[IBIS Ver]   4.2
[File Name]  stm32f2_ufbga176.ibs
[File Rev]   1.0
[Date]   31-Aug-2011
[Source]   STMicroelectronics NV
[Notes]   The I/O models have been made by simulation and qualified
   with recomandation of QualityIBIS flow.
   Some Models, library and pin names may be modified.
   Details of modified names can be found below.
ORIGINAL NAME   ::  MODIFIED NAME   :: COMMENTS(if any)
IO8USB_LSFS_OTG_FT  ::  IO8USB_LSFS_OTG_FT_USB   :: Model in USB mode.
IO8USB_LSFS_OTG_FT  ::  IO8USB_LSFS_OTG_FT_NON_USB_DNV33  :: Model in other than USB mode & pad pin = DNV33
IO8USB_LSFS_OTG_FT  ::  IO8USB_LSFS_OTG_FT_NON_USB_DPV33  :: Model in other than USB mode & pad pin = DPV33
[Disclaimer] These IBIS models are the proprietary information of
   STMicroelectronics and are disclosed to users solely for
   modeling and simulation purposes. No further license is
   implied. All warranties express, implied, or statutory,
   including any implied warranty of fitness for a particular
   purpose or implied warranty against infringement, are
   hereby disclaimed. STMicroelectronics reserves the right
   to change the IBIS models at any time and without notice.
[Copyright]  (c) STMicroelectronics
   All rights reserved. Reproduction in whole or part is prohibited
   without the written consent of the copyright holder.
[Component]  STM32F2_UFBGA176
[Manufacturer] STMicroelectronics NV
[Package]
| variable   typ   min   max
R_pkg   0.000mOhm   0.000mOhm   0.000mOhm
L_pkg   0.000nH   0.000nH   0.000nH
C_pkg   0.000pF   0.000pF   0.000pF
[Pin]   signal_name   model_name
A2 PE2 IO8PROG2M25M50M100M_ARSUDQ_FT
A1 PE3 IO8PROG2M25M50M100M_ARSUDQ_FT
B1 PE4 IO8PROG2M25M50M100M_ARSUDQ_FT
B2 PE5 IO8PROG2M25M50M100M_ARSUDQ_FT
B3 PE6 IO8PROG2M25M50M100M_ARSUDQ_FT
|C1 VBAT VDD33IOSWCO_MOSSWI_FT
D2 PI8 IO8PROG2M25M50M100M_ARSUDQ_FT_V33
D1 PC13 IO8PROG2M25M50M100M_ARWSUDQ_FT_V33
E1 PC14 IO8PROG2M25M50M100M_ARWSUDQ_FT
F1 PC15 IO8PROG2M25M50M100M_ARSUDQ_FT
D3 PI9  IO8PROG2M25M50M100M_ARSUDQ_FT
E3 PI10 IO8PROG2M25M50M100M_ARSUDQ_FT
E4 PI11 IO8PROG2M25M50M100M_ARSUDQ_FT
|F2 VSS_13 VSSIOCO
|F3 VDD_13 VDD33IOCO
E2 PF0 IO8PROG2M25M50M100M_ARSUDQ_FT
H3 PF1 IO8PROG2M25M50M100M_ARSUDQ_FT
H2 PF2 IO8PROG2M25M50M100M_ARSUDQ_FT
J2 PF3 IO8PROG2M25M50M100M_ARSUDQ_FT
J3 PF4 IO8PROG2M25M50M100M_ARSUDQ_FT
K3 PF5 IO8PROG2M25M50M100M_ARSUDQ_FT
|G2 VSS_5 VSSIOCO
|G3 VDD_5 VDD33IOCO
K2 PF6 IO8PROG2M25M50M100M_ARSUDQ_FT
K1 PF7 IO8PROG2M25M50M100M_ARSUDQ_FT
L3 PF8 IO8PROG2M25M50M100M_ARSUDQ_FT
L2 PF9  IO8PROG2M25M50M100M_AR3WSUDQ_FT
L1 PF10 IO8PROG2M25M50M100M_ARSUDQ_FT
G1 PH0 IO8PROG2M25M50M100M_ARSUDQ_FT
H1 PH1 IO8PROG2M25M50M100M_ARSUDQ_FT
|J1 NRST RESET
M2 PC0 IO8PROG2M25M50M100M_AR3WSUDQ_FT
M3 PC1 IO8PROG2M25M50M100M_AR3WSUDQ_FT
M4 PC2 IO8PROG2M25M50M100M_AR3WSUDQ_FT
M5 PC3 IO8PROG2M25M50M100M_AR3WSUDQ_FT
|- VDD_12 VDD33IOCO_VSSIOCO_MOSSWI_FT
|M1 VSSA VSSCO
|N1 VREF- VSSC0
|P1 VREF+ VDD33CO
|R1 VDDA VDD33CO
N3 PA0 IO8PROG2M25M50M100M_AR3WSUDQ_FT_V33
N2 PA1 IO8PROG2M25M50M100M_AR3WSUDQ_FT
P2 PA2 IO8PROG2M25M50M100M_AR3WSUDQ_FT
F4 PH2 IO8PROG2M25M50M100M_AR3WSUDQ_FT
G4 PH3 IO8PROG2M25M50M100M_AR3WSUDQ_FT
H4 PH4 IO8PROG2M25M50M100M_AR3WSUDQ_FT
J4 PH5 IO8PROG2M25M50M100M_AR3WSUDQ_FT
R2 PA3 IO8PROG2M25M50M100M_AR3WSUDQ_FT
|- VSS_4 VSSIOCO
|L4 REGOFF   TBD
|K4 VDD_4 VDD33IOCO
N4 PA4 IO8PROG2M25M50M100M_AR3WSUDQ_FT
P4 PA5 IO8PROG2M25M50M100M_AR3WSUDQ_FT
P3 PA6 IO8PROG2M25M50M100M_AR3WSUDQ_FT
R3 PA7 IO8PROG2M25M50M100M_AR3WSUDQ_FT
N5 PC4 IO8PROG2M25M50M100M_AR3WSUDQ_FT
P5 PC5 IO8PROG2M25M50M100M_AR3WSUDQ_FT
R5 PB0 IO8PROG2M25M50M100M_AR3WSUDQ_FT
R4 PB1 IO8PROG2M25M50M100M_AR3WSUDQ_FT
M6 PB2 IO8PROG2M25M50M100M_AR3WSUDQ_FT
R6 PF11 IO8PROG2M25M50M100M_ARSUDQ_FT
P6 PF12 IO8PROG2M25M50M100M_ARSUDQ_FT
|M8 VSS_6 VSSIOCO
|N8 VDD_6 VDD33IOCO
N6 PF13 IO8PROG2M25M50M100M_ARSUDQ_FT
R7 PF14 IO8PROG2M25M50M100M_ARSUDQ_FT
P7 PF15 IO8PROG2M25M50M100M_ARSUDQ_FT
N7 PG0 IO8PROG2M25M50M100M_ARSUDQ_FT
M7 PG1 IO8PROG2M25M50M100M_ARSUDQ_FT
R8 PE7 IO8PROG2M25M50M100M_ARSUDQ_FT
P8 PE8 IO8PROG2M25M50M100M_ARSUDQ_FT
P9 PE9 IO8PROG2M25M50M100M_ARSUDQ_FT
|M9 VSS_7 VSSIOCO
|N9 VDD_7 VDD33IOCO
R9 PE10 IO8PROG2M25M50M100M_ARSUDQ_FT
P10 PE11 IO8PROG2M25M50M100M_ARSUDQ_FT
R10 PE12 IO8PROG2M25M50M100M_ARSUDQ_FT
N11 PE13 IO8PROG2M25M50M100M_ARSUDQ_FT
P11 PE14 IO8PROG2M25M50M100M_ARSUDQ_FT
R11 PE15 IO8PROG2M25M50M100M_ARSUDQ_FT
R12 PB10 IO8PROG2M25M50M100M_ARSUDQ_I2CIN_FT
R13 PB11 IO8PROG2M25M50M100M_ARSUDQ_I2CIN_FT
|M10 VCAP_1
|N10 VDD_1 VDD33IOCO
M11 PH6 IO8PROG2M25M50M100M_ARSUDQ_FT
N12 PH7 IO8PROG2M25M50M100M_ARSUDQ_FT
M12 PH8 IO8PROG2M25M50M100M_ARSUDQ_FT
M13 PH9 IO8PROG2M25M50M100M_ARSUDQ_FT
L13 PH10 IO8PROG2M25M50M100M_ARSUDQ_FT
L12 PH11 IO8PROG2M25M50M100M_ARSUDQ_FT
K12 PH12 IO8PROG2M25M50M100M_ARSUDQ_FT
|H12 VSS_14 VSSIOCO
|J12 VDD_14 VDD33IOCO
P12 PB12 IO8USB_ID_OTG_FT
P13 PB13 IO8USB_VBUS_OTG_FT
R14 PB14 IO8USB_LSFS_OTG_FT_USB
|R14 PB14 IO8USB_LSFS_OTG_FT_NON_USB_DNV33
R15 PB15 IO8USB_LSFS_OTG_FT_USB
|R15 PB15 IO8USB_LSFS_OTG_FT_NON_USB_DPV3394
P15 PD8 IO8PROG2M25M50M100M_ARSUDQ_FT
P14 PD9 IO8PROG2M25M50M100M_ARSUDQ_FT
N15 PD10 IO8PROG2M25M50M100M_ARSUDQ_FT
N14 PD11 IO8PROG2M25M50M100M_ARSUDQ_FT
N13 PD12 IO8PROG2M25M50M100M_ARSUDQ_FT
M15 PD13 IO8PROG2M25M50M100M_ARSUDQ_FT
|- VSS_8 VSSIOCO
|J13 VDD_8 VDD33IOCO
M14 PD14 IO8PROG2M25M50M100M_ARSUDQ_FT
L14 PD15 IO8PROG2M25M50M100M_ARSUDQ_FT
L15 PG2 IO8PROG2M25M50M100M_ARSUDQ_FT
K15 PG3 IO8PROG2M25M50M100M_ARSUDQ_FT
K14 PG4 IO8PROG2M25M50M100M_ARSUDQ_FT
K13 PG5 IO8PROG2M25M50M100M_ARSUDQ_FT
J15 PG6 IO8PROG2M25M50M100M_ARSUDQ_FT
J14 PG7 IO8PROG2M25M50M100M_ARSUDQ_FT
H14 PG8 IO8PROG2M25M50M100M_ARSUDQ_FT
|G12 VSS_9 VSSIOCO
|H13 VDD_9 VDD33IOCO
H15 PC6 IO8PROG2M25M50M100M_ARSUDQ_FT
G15 PC7 IO8PROG2M25M50M100M_ARSUDQ_FT
G14 PC8 IO8PROG2M25M50M100M_ARSUDQ_FT
F14 PC9 IO8PROG2M25M50M100M_ARSUDQ_I2CIN_FT
F15 PA8 IO8PROG2M25M50M100M_ARSUDQ_I2CIN_FT
E15 PA9 IO8USB_VBUS_OTG_FT
D15 PA10 IO8USB_ID_OTG_FT
|C15 PA11 IO8USB_LSFS_OTG_FT_USB
C15 PA11 IO8USB_LSFS_OTG_FT_NON_USB_DNV33
|B15 PA12 IO8USB_LSFS_OTG_FT_USB
B15 PA12 IO8USB_LSFS_OTG_FT_NON_USB_DPV33
A15 PA13 IO8PROG2M25M50M100M_ARSUDQ_FT
|F13 VCAP_2
|F12 VSS_2 VSSIOCO
|G13 VDD_2 VDD33IOCO
E12 PH13 IO8PROG2M25M50M100M_ARSUDQ_FT
E13 PH14 IO8PROG2M25M50M100M_ARSUDQ_FT
D13 PH15 IO8PROG2M25M50M100M_ARSUDQ_FT
E14 PI0 IO8PROG2M25M50M100M_ARSUDQ_FT
D14 PI1 IO8PROG2M25M50M100M_ARSUDQ_FT
C14 PI2 IO8PROG2M25M50M100M_ARSUDQ_FT
C13 PI3 IO8PROG2M25M50M100M_ARSUDQ_FT
|D9 VSS_15 VSSIOCO
|C9 VDD_15 VDD33IOCO
A14 PA14 IO8PROG2M25M50M100M_ARSUDQ_FT
A13 PA15 IO8PROG2M25M50M100M_AR3WSUDQ_FT
B14 PC10 IO8PROG2M25M50M100M_ARSUDQ_FT
B13 PC11 IO8PROG2M25M50M100M_ARSUDQ_FT
A12 PC12 IO8PROG2M25M50M100M_ARSUDQ_FT
B12 PD0 IO8PROG2M25M50M100M_ARSUDQ_FT
C12 PD1 IO8PROG2M25M50M100M_ARSUDQ_FT
D12 PD2 IO8PROG2M25M50M100M_ARSUDQ_FT
D11 PD3 IO8PROG2M25M50M100M_ARSUDQ_FT
D10 PD4 IO8PROG2M25M50M100M_ARSUDQ_FT
C11 PD5 IO8PROG2M25M50M100M_ARSUDQ_FT
|D8 VSS_10 VSSIOCO
|C8 VDD_10 VDD33IOCO
B11 PD6 IO8PROG2M25M50M100M_ARSUDQ_FT
A11 PD7 IO8PROG2M25M50M100M_ARSUDQ_FT
C10 PG9 IO8PROG2M25M50M100M_ARSUDQ_FT
B10 PG10 IO8PROG2M25M50M100M_ARSUDQ_FT
B9 PG11 IO8PROG2M25M50M100M_ARSUDQ_FT
B8 PG12 IO8PROG2M25M50M100M_ARSUDQ_FT
A8 PG13 IO8PROG2M25M50M100M_ARSUDQ_FT
A7 PG14 IO8PROG2M25M50M100M_ARSUDQ_FT
|D7 VSS_11 VSSIOCO
|C7 VDD_11 VDD33IOCO
B7 PG15 IO8PROG2M25M50M100M_ARSUDQ_FT
A10 PB3 IO8PROG2M25M50M100M_ARSUDQ_FT
A9 PB4 IO8PROG2M25M50M100M_ARSUDQ_FT
A6 PB5 IO8PROG2M25M50M100M_AR3WSUDQ_FT
B6 PB6 IO8PROG2M25M50M100M_ARSUDQ_I2CIN_FT
B5 PB7 IO8PROG2M25M50M100M_ARSUDQ_I2CIN_FT
D6 BOOT0 VPP_TEST_HV
A5 PB8 IO8PROG2M25M50M100M_ARSUDQ_I2CIN_FT
B4 PB9 IO8PROG2M25M50M100M_ARSUDQ_I2CIN_FT
A4 PE0 IO8PROG2M25M50M100M_ARSUDQ_FT
A3 PE1 IO8PROG2M25M50M100M_ARSUDQ_FT
|D5 VSS VSSIOCO
|C6 RFU VDD33IOCO
|C5 VDD_3 VDD33IOCO
D4 PI4 IO8PROG2M25M50M100M_ARSUDQ_FT
C4 PI5 IO8PROG2M25M50M100M_ARSUDQ_FT
C3 PI6 IO8PROG2M25M50M100M_ARSUDQ_FT
C2 PI7 IO8PROG2M25M50M100M_ARSUDQ_FT
[Diff Pin]  inv_pin   vdiff tdelay_typ tdelay_min tdelay_max
R14 R15 200mV 0  0 0
C15 B15 200mV 0  0 0
[Model Selector] IO8PROG2M25M50M100M_ARSUDQ_FT_V33
IO8PROG2M25M50M100M_ARSUDQ_DRV_V33_00   DRIVER MODEL  : SPEEDAV33=0 SPEEDBV33=0
IO8PROG2M25M50M100M_ARSUDQ_DRV_V33_01   DRIVER MODEL  : SPEEDAV33=0 SPEEDBV33=1
IO8PROG2M25M50M100M_ARSUDQ_DRV_V33_10   DRIVER MODEL  : SPEEDAV33=1 SPEEDBV33=0
IO8PROG2M25M50M100M_ARSUDQ_DRV_V33_11   DRIVER MODEL  : SPEEDAV33=1 SPEEDBV33=1
IO8PROG2M25M50M100M_ARSUDQ_RCV_V33_0   CMOS RECIEVER : ENHYSV33=0  OUTPUT=ZIV33
IO8PROG2M25M50M100M_ARSUDQ_RCV_V33_0_T   TTL  RECIEVER : ENHYSV33=0  OUTPUT=ZIV33
IO8PROG2M25M50M100M_ARSUDQ_RCV_V33_1   CMOS RECIEVER : ENHYSV33=1  OUTPUT=ZIV33
IO8PROG2M25M50M100M_ARSUDQ_RCV_V33_1_T   TTL  RECIEVER : ENHYSV33=1  OUTPUT=ZIV33
[Model Selector] IO8PROG2M25M50M100M_AR3WSUDQ_FT_V33
IO8PROG2M25M50M100M_AR3WSUDQ_DRV_V33_00   DRIVER MODEL  : SPEEDAV33=0 SPEEDBV33=0
IO8PROG2M25M50M100M_AR3WSUDQ_DRV_V33_01   DRIVER MODEL  : SPEEDAV33=0 SPEEDBV33=1
IO8PROG2M25M50M100M_AR3WSUDQ_DRV_V33_10   DRIVER MODEL  : SPEEDAV33=1 SPEEDBV33=0
IO8PROG2M25M50M100M_AR3WSUDQ_DRV_V33_11   DRIVER MODEL  : SPEEDAV33=1 SPEEDBV33=1
IO8PROG2M25M50M100M_AR3WSUDQ_RCV_V33_0   CMOS RECIEVER : ENHYSV33=0  OUTPUT=ZIV33
IO8PROG2M25M50M100M_AR3WSUDQ_RCV_V33_0_T  TTL  RECIEVER : ENHYSV33=0  OUTPUT=ZIV33
IO8PROG2M25M50M100M_AR3WSUDQ_RCV_V33_1   CMOS RECIEVER : ENHYSV33=1  OUTPUT=ZIV33
IO8PROG2M25M50M100M_AR3WSUDQ_RCV_V33_1_T  TTL  RECIEVER : ENHYSV33=1  OUTPUT=ZIV33
[Model Selector] IO8PROG2M25M50M100M_AR3WSUDQ_FT
IO8PROG2M25M50M100M_AR3WSUDQ_FT_DRV_00   DRIVER MODEL  : SPEEDAV12=0 SPEEDBV12=0
IO8PROG2M25M50M100M_AR3WSUDQ_FT_DRV_01   DRIVER MODEL  : SPEEDAV12=0 SPEEDBV12=1
IO8PROG2M25M50M100M_AR3WSUDQ_FT_DRV_10   DRIVER MODEL  : SPEEDAV12=1 SPEEDBV12=0
IO8PROG2M25M50M100M_AR3WSUDQ_FT_DRV_11   DRIVER MODEL  : SPEEDAV12=1 SPEEDBV12=1
IO8PROG2M25M50M100M_AR3WSUDQ_FT_RCV_00   CMOS RECIEVER : ENHYSV12=0  OUTPUT=ZIV12
IO8PROG2M25M50M100M_AR3WSUDQ_FT_RCV_00_T  TTL  RECIEVER : ENHYSV12=0  OUTPUT=ZIV12
IO8PROG2M25M50M100M_AR3WSUDQ_FT_RCV_01   CMOS RECIEVER : ENHYSV12=0  OUTPUT=ZIV33
IO8PROG2M25M50M100M_AR3WSUDQ_FT_RCV_01_T  TTL  RECIEVER : ENHYSV12=0  OUTPUT=ZIV33
IO8PROG2M25M50M100M_AR3WSUDQ_FT_RCV_10   CMOS RECIEVER : ENHYSV12=1  OUTPUT=ZIV12
IO8PROG2M25M50M100M_AR3WSUDQ_FT_RCV_10_T  TTL  RECIEVER : ENHYSV12=1  OUTPUT=ZIV12
IO8PROG2M25M50M100M_AR3WSUDQ_FT_RCV_11   CMOS RECIEVER : ENHYSV12=1  OUTPUT=ZIV33
IO8PROG2M25M50M100M_AR3WSUDQ_FT_RCV_11_T  TTL  RECIEVER : ENHYSV12=1  OUTPUT=ZIV33
[Model Selector] IO8PROG2M25M50M100M_ARSUDQ_FT
IO8PROG2M25M50M100M_ARSUDQ_FT_DRV_00   DRIVER MODEL  : SPEEDAV12=0 SPEEDBV12=0
IO8PROG2M25M50M100M_ARSUDQ_FT_DRV_01   DRIVER MODEL  : SPEEDAV12=0 SPEEDBV12=1
IO8PROG2M25M50M100M_ARSUDQ_FT_DRV_10   DRIVER MODEL  : SPEEDAV12=1 SPEEDBV12=0
IO8PROG2M25M50M100M_ARSUDQ_FT_DRV_11   DRIVER MODEL  : SPEEDAV12=1 SPEEDBV12=1
IO8PROG2M25M50M100M_ARSUDQ_FT_RCV_00   CMOS RECIEVER : ENHYSV12=0  OUTPUT=ZIV12
IO8PROG2M25M50M100M_ARSUDQ_FT_RCV_00_T   TTL  RECIEVER : ENHYSV12=0  OUTPUT=ZIV12
IO8PROG2M25M50M100M_ARSUDQ_FT_RCV_01   CMOS RECIEVER : ENHYSV12=0  OUTPUT=ZIV33
IO8PROG2M25M50M100M_ARSUDQ_FT_RCV_01_T   TTL  RECIEVER : ENHYSV12=0  OUTPUT=ZIV33
IO8PROG2M25M50M100M_ARSUDQ_FT_RCV_10   CMOS RECIEVER : ENHYSV12=1  OUTPUT=ZIV12
IO8PROG2M25M50M100M_ARSUDQ_FT_RCV_10_T   TTL  RECIEVER : ENHYSV12=1  OUTPUT=ZIV12
IO8PROG2M25M50M100M_ARSUDQ_FT_RCV_11   CMOS RECIEVER : ENHYSV12=1  OUTPUT=ZIV33
IO8PROG2M25M50M100M_ARSUDQ_FT_RCV_11_T   TTL  RECIEVER : ENHYSV12=1  OUTPUT=ZIV33
[Model Selector] IO8PROG2M25M50M100M_ARSUDQ_I2CIN_FT
IO8PROG2M25M50M100M_ARSUDQ_I2CIN_DRV_00   DRIVER MODEL  : SPEEDAV12=0 SPEEDBV12=0
IO8PROG2M25M50M100M_ARSUDQ_I2CIN_DRV_01   DRIVER MODEL  : SPEEDAV12=0 SPEEDBV12=1
IO8PROG2M25M50M100M_ARSUDQ_I2CIN_DRV_10   DRIVER MODEL  : SPEEDAV12=1 SPEEDBV12=0
IO8PROG2M25M50M100M_ARSUDQ_I2CIN_DRV_11   DRIVER MODEL  : SPEEDAV12=1 SPEEDBV12=1
IO8PROG2M25M50M100M_I2CIN_RCV_ZII2C_00   CMOS RECIEVER : TESTI2CV12=0  HSFSV12=0
IO8PROG2M25M50M100M_I2CIN_RCV_ZII2C_00_T   TTL  RECIEVER : TESTI2CV12=0  HSFSV12=0
IO8PROG2M25M50M100M_I2CIN_RCV_ZII2C_01   CMOS RECIEVER : TESTI2CV12=0  HSFSV12=1
IO8PROG2M25M50M100M_I2CIN_RCV_ZII2C_01_T   TTL  RECIEVER : TESTI2CV12=0  HSFSV12=1
IO8PROG2M25M50M100M_I2CIN_RCV_ZII2C_10   CMOS RECIEVER : TESTI2CV12=1  HSFSV12=0
IO8PROG2M25M50M100M_I2CIN_RCV_ZII2C_10_T   TTL  RECIEVER : TESTI2CV12=1  HSFSV12=0
IO8PROG2M25M50M100M_I2CIN_RCV_ZII2C_11   CMOS RECIEVER : TESTI2CV12=1  HSFSV12=1
IO8PROG2M25M50M100M_I2CIN_RCV_ZII2C_11_T   TTL  RECIEVER : TESTI2CV12=1  HSFSV12=1
IO8PROG2M25M50M100M_I2CIN_RCV_ZIV12_0   CMOS RECIEVER : ENHYSV12=0  OUTPUT=ZIV12
IO8PROG2M25M50M100M_I2CIN_RCV_ZIV12_0_T   TTL  RECIEVER : ENHYSV12=0  OUTPUT=ZIV12
IO8PROG2M25M50M100M_I2CIN_RCV_ZIV12_1   CMOS RECIEVER : ENHYSV12=1  OUTPUT=ZIV12
IO8PROG2M25M50M100M_I2CIN_RCV_ZIV12_1_T   TTL  RECIEVER : ENHYSV12=1  OUTPUT=ZIV12
IO8PROG2M25M50M100M_I2CIN_RCV_ZIV33_0   CMOS RECIEVER : ENHYSV12=0  OUTPUT=ZIV33
IO8PROG2M25M50M100M_I2CIN_RCV_ZIV33_0_T   TTL  RECIEVER : ENHYSV12=0  OUTPUT=ZIV33
IO8PROG2M25M50M100M_I2CIN_RCV_ZIV33_1   CMOS RECIEVER : ENHYSV12=1  OUTPUT=ZIV33
IO8PROG2M25M50M100M_I2CIN_RCV_ZIV33_1_T   TTL  RECIEVER : ENHYSV12=1  OUTPUT=ZIV33
[Model Selector] IO8PROG2M25M50M100M_ARWSUDQ_FT_V33
IO8PROG2M25M50M100M_ARWSUDQ_DRV_V33_00   DRIVER MODEL  : SPEEDAV33=0 SPEEDBV33=0
IO8PROG2M25M50M100M_ARWSUDQ_DRV_V33_01   DRIVER MODEL  : SPEEDAV33=0 SPEEDBV33=1
IO8PROG2M25M50M100M_ARWSUDQ_DRV_V33_10   DRIVER MODEL  : SPEEDAV33=1 SPEEDBV33=0
IO8PROG2M25M50M100M_ARWSUDQ_DRV_V33_11   DRIVER MODEL  : SPEEDAV33=1 SPEEDBV33=1
IO8PROG2M25M50M100M_ARWSUDQ_RCV_V33_0   CMOS RECIEVER : ENHYSV33=0  OUTPUT=ZIV33
IO8PROG2M25M50M100M_ARWSUDQ_RCV_V33_0_T   TTL  RECIEVER : ENHYSV33=0  OUTPUT=ZIV33
IO8PROG2M25M50M100M_ARWSUDQ_RCV_V33_1   CMOS RECIEVER : ENHYSV33=1  OUTPUT=ZIV33
IO8PROG2M25M50M100M_ARWSUDQ_RCV_V33_1_T   TTL  RECIEVER : ENHYSV33=1  OUTPUT=ZIV33
[Model Selector] IO8PROG2M25M50M100M_ARWSUDQ_FT
IO8PROG2M25M50M100M_ARWSUDQ_FT_DRV_00   DRIVER MODEL  : SPEEDAV12=0 SPEEDBV12=0
IO8PROG2M25M50M100M_ARWSUDQ_FT_DRV_01   DRIVER MODEL  : SPEEDAV12=0 SPEEDBV12=1
IO8PROG2M25M50M100M_ARWSUDQ_FT_DRV_10   DRIVER MODEL  : SPEEDAV12=1 SPEEDBV12=0
IO8PROG2M25M50M100M_ARWSUDQ_FT_DRV_11   DRIVER MODEL  : SPEEDAV12=1 SPEEDBV12=1
IO8PROG2M25M50M100M_ARWSUDQ_FT_RCV_00   CMOS RECIEVER : ENHYSV12=0  OUTPUT=ZIV12
IO8PROG2M25M50M100M_ARWSUDQ_FT_RCV_00_T   TTL  RECIEVER : ENHYSV12=0  OUTPUT=ZIV12
IO8PROG2M25M50M100M_ARWSUDQ_FT_RCV_01   CMOS RECIEVER : ENHYSV12=0  OUTPUT=ZIV33
IO8PROG2M25M50M100M_ARWSUDQ_FT_RCV_01_T   TTL  RECIEVER : ENHYSV12=0  OUTPUT=ZIV33
IO8PROG2M25M50M100M_ARWSUDQ_FT_RCV_10   CMOS RECIEVER : ENHYSV12=1  OUTPUT=ZIV12
IO8PROG2M25M50M100M_ARWSUDQ_FT_RCV_10_T   TTL  RECIEVER : ENHYSV12=1  OUTPUT=ZIV12
IO8PROG2M25M50M100M_ARWSUDQ_FT_RCV_11   CMOS RECIEVER : ENHYSV12=1  OUTPUT=ZIV33
IO8PROG2M25M50M100M_ARWSUDQ_FT_RCV_11_T   TTL  RECIEVER : ENHYSV12=1  OUTPUT=ZIV33
[Model Selector] IO8USB_ID_OTG_FT
IO8USB_ID_OTG_FT_DRV_00   DRIVER MODEL  : SPEEDAV12=0 SPEEDBV12=0
IO8USB_ID_OTG_FT_DRV_01   DRIVER MODEL  : SPEEDAV12=0 SPEEDBV12=1
IO8USB_ID_OTG_FT_DRV_10   DRIVER MODEL  : SPEEDAV12=1 SPEEDBV12=0
IO8USB_ID_OTG_FT_DRV_11   DRIVER MODEL  : SPEEDAV12=1 SPEEDBV12=1
IO8USB_ID_OTG_FT_RCV_00   CMOS RECIEVER : ENHYSV12=0  OUTPUT=ZIV12
IO8USB_ID_OTG_FT_RCV_00_T   TTL  RECIEVER : ENHYSV12=0  OUTPUT=ZIV12
IO8USB_ID_OTG_FT_RCV_01   CMOS RECIEVER : ENHYSV12=0  OUTPUT=ZIV33
IO8USB_ID_OTG_FT_RCV_01_T   TTL  RECIEVER : ENHYSV12=0  OUTPUT=ZIV33
IO8USB_ID_OTG_FT_RCV_10   CMOS RECIEVER : ENHYSV12=1  OUTPUT=ZIV12
IO8USB_ID_OTG_FT_RCV_10_T   TTL  RECIEVER : ENHYSV12=1  OUTPUT=ZIV12
IO8USB_ID_OTG_FT_RCV_11   CMOS RECIEVER : ENHYSV12=1  OUTPUT=ZIV33
IO8USB_ID_OTG_FT_RCV_11_T   TTL  RECIEVER : ENHYSV12=1  OUTPUT=ZIV33
[Model Selector] IO8USB_LSFS_OTG_FT_USB
IO8USB_LSFS_OTG_FT_DRV_USB_0   DRIVER : USBLSFSV12=0 ENUSBV12=0
IO8USB_LSFS_OTG_FT_DRV_USB_1   DRIVER : USBLSFSV12=1 ENUSBV12=0
IO8USB_LSFS_OTG_FT_RCV_USB   USB  RECIEVER : ENHYSV12=1  OUTPUT=USBZIV12
[Model Selector] IO8USB_LSFS_OTG_FT_NON_USB_DNV33
IO8USB_LSFS_OTG_FT_DRV_IO8_DNV33_00   DRIVER : SPEEDAV12=0 SPEEDBV12=0 ENUSBV12=1
IO8USB_LSFS_OTG_FT_DRV_IO8_DNV33_01   DRIVER : SPEEDAV12=0 SPEEDBV12=1 ENUSBV12=1
IO8USB_LSFS_OTG_FT_DRV_IO8_DNV33_10   DRIVER : SPEEDAV12=1 SPEEDBV12=0 ENUSBV12=1
IO8USB_LSFS_OTG_FT_DRV_IO8_DNV33_11   DRIVER : SPEEDAV12=1 SPEEDBV12=1 ENUSBV12=1
IO8USB_LSFS_OTG_FT_RCV_IO8_ZINV12_0   CMOS RECIEVER : ENHYSV12=0  OUTPUT=ZIV12
IO8USB_LSFS_OTG_FT_RCV_IO8_ZINV12_0_T  TTL  RECIEVER : ENHYSV12=0  OUTPUT=ZIV12
IO8USB_LSFS_OTG_FT_RCV_IO8_ZINV12_1   CMOS RECIEVER : ENHYSV12=1  OUTPUT=ZIV12
IO8USB_LSFS_OTG_FT_RCV_IO8_ZINV12_1_T  TTL  RECIEVER : ENHYSV12=1  OUTPUT=ZIV12
IO8USB_LSFS_OTG_FT_RCV_IO8_ZINV33_0   CMOS RECIEVER : ENHYSV12=0  OUTPUT=ZIV33
IO8USB_LSFS_OTG_FT_RCV_IO8_ZINV33_0_T  TTL  RECIEVER : ENHYSV12=0  OUTPUT=ZIV33
IO8USB_LSFS_OTG_FT_RCV_IO8_ZINV33_1   CMOS RECIEVER : ENHYSV12=1  OUTPUT=ZIV33
IO8USB_LSFS_OTG_FT_RCV_IO8_ZINV33_1_T  TTL  RECIEVER : ENHYSV12=1  OUTPUT=ZIV33
[Model Selector] IO8USB_LSFS_OTG_FT_NON_USB_DPV33
IO8USB_LSFS_OTG_FT_DRV_IO8_DPV33_00   DRIVER : SPEEDAV12=0 SPEEDBV12=0 ENUSBV12=1
IO8USB_LSFS_OTG_FT_DRV_IO8_DPV33_01   DRIVER : SPEEDAV12=0 SPEEDBV12=1 ENUSBV12=1
IO8USB_LSFS_OTG_FT_DRV_IO8_DPV33_10   DRIVER : SPEEDAV12=1 SPEEDBV12=0 ENUSBV12=1
IO8USB_LSFS_OTG_FT_DRV_IO8_DPV33_11   DRIVER : SPEEDAV12=1 SPEEDBV12=1 ENUSBV12=1
IO8USB_LSFS_OTG_FT_RCV_IO8_ZIPV12_0   CMOS RECIEVER : ENHYSV12=0  OUTPUT=ZIV12
IO8USB_LSFS_OTG_FT_RCV_IO8_ZIPV12_0_T  TTL  RECIEVER : ENHYSV12=0  OUTPUT=ZIV12
IO8USB_LSFS_OTG_FT_RCV_IO8_ZIPV12_1   CMOS RECIEVER : ENHYSV12=1  OUTPUT=ZIV12
IO8USB_LSFS_OTG_FT_RCV_IO8_ZIPV12_1_T  TTL  RECIEVER : ENHYSV12=1  OUTPUT=ZIV12
IO8USB_LSFS_OTG_FT_RCV_IO8_ZIPV33_0   CMOS RECIEVER : ENHYSV12=0  OUTPUT=ZIV33
IO8USB_LSFS_OTG_FT_RCV_IO8_ZIPV33_0_T  TTL  RECIEVER : ENHYSV12=0  OUTPUT=ZIV33
IO8USB_LSFS_OTG_FT_RCV_IO8_ZIPV33_1   CMOS RECIEVER : ENHYSV12=1  OUTPUT=ZIV33
IO8USB_LSFS_OTG_FT_RCV_IO8_ZIPV33_1_T  TTL  RECIEVER : ENHYSV12=1  OUTPUT=ZIV33
[Model Selector] IO8USB_VBUS_OTG_FT
IO8USB_VBUS_OTG_FT_DRV_00   DRIVER MODEL  : SPEEDAV12=0 SPEEDBV12=0
IO8USB_VBUS_OTG_FT_DRV_01   DRIVER MODEL  : SPEEDAV12=0 SPEEDBV12=1
IO8USB_VBUS_OTG_FT_DRV_10   DRIVER MODEL  : SPEEDAV12=1 SPEEDBV12=0
IO8USB_VBUS_OTG_FT_DRV_11   DRIVER MODEL  : SPEEDAV12=1 SPEEDBV12=1
IO8USB_VBUS_OTG_FT_RCV_00   CMOS RECIEVER : ENHYSV12=0  OUTPUT=ZIV12
IO8USB_VBUS_OTG_FT_RCV_00_T   TTL  RECIEVER : ENHYSV12=0  OUTPUT=ZIV12
IO8USB_VBUS_OTG_FT_RCV_01   CMOS RECIEVER : ENHYSV12=0  OUTPUT=ZIV33
IO8USB_VBUS_OTG_FT_RCV_01_T   TTL  RECIEVER : ENHYSV12=0  OUTPUT=ZIV33
IO8USB_VBUS_OTG_FT_RCV_10   CMOS RECIEVER : ENHYSV12=1  OUTPUT=ZIV12
IO8USB_VBUS_OTG_FT_RCV_10_T   TTL  RECIEVER : ENHYSV12=1  OUTPUT=ZIV12
IO8USB_VBUS_OTG_FT_RCV_11   CMOS RECIEVER : ENHYSV12=1  OUTPUT=ZIV33
IO8USB_VBUS_OTG_FT_RCV_11_T   TTL  RECIEVER : ENHYSV12=1  OUTPUT=ZIV33
[Model Selector] VPP_TEST_HV
VPP_TEST_HV_00   CMOS RECIEVER : ENHYSV12=0  OUTPUT=ZIV12
VPP_TEST_HV_00_T   TTL  RECIEVER : ENHYSV12=0  OUTPUT=ZIV12
VPP_TEST_HV_01   CMOS RECIEVER : ENHYSV12=0  OUTPUT=ZIV33
VPP_TEST_HV_01_T   TTL  RECIEVER : ENHYSV12=0  OUTPUT=ZIV33
VPP_TEST_HV_10   CMOS RECIEVER : ENHYSV12=1  OUTPUT=ZIV12
VPP_TEST_HV_10_T   TTL  RECIEVER : ENHYSV12=1  OUTPUT=ZIV12
VPP_TEST_HV_11   CMOS RECIEVER : ENHYSV12=1  OUTPUT=ZIV33
VPP_TEST_HV_11_T   TTL  RECIEVER : ENHYSV12=1  OUTPUT=ZIV33
| Models and submodels in the file (139): IO8PROG2M25M50M100M_AR3WSUDQ_DRV_V33_00 (3-state), IO8PROG2M25M50M100M_AR3WSUDQ_DRV_V33_01 (3-state), IO8PROG2M25M50M100M_AR3WSUDQ_DRV_V33_10 (3-state), IO8PROG2M25M50M100M_AR3WSUDQ_DRV_V33_11 (3-state), IO8PROG2M25M50M100M_AR3WSUDQ_FT_DRV_00 (3-state), IO8PROG2M25M50M100M_AR3WSUDQ_FT_DRV_01 (3-state), IO8PROG2M25M50M100M_AR3WSUDQ_FT_DRV_10 (3-state), IO8PROG2M25M50M100M_AR3WSUDQ_FT_DRV_11 (3-state), IO8PROG2M25M50M100M_AR3WSUDQ_FT_RCV_00 (Input), IO8PROG2M25M50M100M_AR3WSUDQ_FT_RCV_00_T (Input), IO8PROG2M25M50M100M_AR3WSUDQ_FT_RCV_01 (Input), IO8PROG2M25M50M100M_AR3WSUDQ_FT_RCV_01_T (Input), IO8PROG2M25M50M100M_AR3WSUDQ_FT_RCV_10 (Input), IO8PROG2M25M50M100M_AR3WSUDQ_FT_RCV_10_T (Input), IO8PROG2M25M50M100M_AR3WSUDQ_FT_RCV_11 (Input), IO8PROG2M25M50M100M_AR3WSUDQ_FT_RCV_11_T (Input), IO8PROG2M25M50M100M_AR3WSUDQ_RCV_V33_0 (Input), IO8PROG2M25M50M100M_AR3WSUDQ_RCV_V33_0_T (Input), IO8PROG2M25M50M100M_AR3WSUDQ_RCV_V33_1 (Input), IO8PROG2M25M50M100M_AR3WSUDQ_RCV_V33_1_T (Input), IO8PROG2M25M50M100M_ARSUDQ_FT_DRV_00 (3-state), IO8PROG2M25M50M100M_ARSUDQ_FT_DRV_01 (3-state), IO8PROG2M25M50M100M_ARSUDQ_FT_DRV_10 (3-state), IO8PROG2M25M50M100M_ARSUDQ_FT_DRV_11 (3-state), IO8PROG2M25M50M100M_ARSUDQ_FT_RCV_00 (Input), IO8PROG2M25M50M100M_ARSUDQ_FT_RCV_00_T (Input), IO8PROG2M25M50M100M_ARSUDQ_FT_RCV_01 (Input), IO8PROG2M25M50M100M_ARSUDQ_FT_RCV_01_T (Input), IO8PROG2M25M50M100M_ARSUDQ_FT_RCV_10 (Input), IO8PROG2M25M50M100M_ARSUDQ_FT_RCV_10_T (Input), IO8PROG2M25M50M100M_ARSUDQ_FT_RCV_11 (Input), IO8PROG2M25M50M100M_ARSUDQ_FT_RCV_11_T (Input), IO8PROG2M25M50M100M_ARSUDQ_I2CIN_DRV_00 (3-state), IO8PROG2M25M50M100M_ARSUDQ_I2CIN_DRV_01 (3-state), IO8PROG2M25M50M100M_ARSUDQ_I2CIN_DRV_10 (3-state), IO8PROG2M25M50M100M_ARSUDQ_I2CIN_DRV_11 (3-state), IO8PROG2M25M50M100M_ARWSUDQ_DRV_V33_00 (3-state), IO8PROG2M25M50M100M_ARWSUDQ_DRV_V33_01 (3-state), IO8PROG2M25M50M100M_ARWSUDQ_DRV_V33_10 (3-state), IO8PROG2M25M50M100M_ARWSUDQ_DRV_V33_11 (3-state), IO8PROG2M25M50M100M_ARWSUDQ_FT_DRV_00 (3-state), IO8PROG2M25M50M100M_ARWSUDQ_FT_DRV_01 (3-state), IO8PROG2M25M50M100M_ARWSUDQ_FT_DRV_10 (3-state), IO8PROG2M25M50M100M_ARWSUDQ_FT_DRV_11 (3-state), IO8PROG2M25M50M100M_ARWSUDQ_FT_RCV_00 (Input), IO8PROG2M25M50M100M_ARWSUDQ_FT_RCV_00_T (Input), IO8PROG2M25M50M100M_ARWSUDQ_FT_RCV_01 (Input), IO8PROG2M25M50M100M_ARWSUDQ_FT_RCV_01_T (Input), IO8PROG2M25M50M100M_ARWSUDQ_FT_RCV_10 (Input), IO8PROG2M25M50M100M_ARWSUDQ_FT_RCV_10_T (Input), IO8PROG2M25M50M100M_ARWSUDQ_FT_RCV_11 (Input), IO8PROG2M25M50M100M_ARWSUDQ_FT_RCV_11_T (Input), IO8PROG2M25M50M100M_ARWSUDQ_RCV_V33_0 (Input), IO8PROG2M25M50M100M_ARWSUDQ_RCV_V33_0_T (Input), IO8PROG2M25M50M100M_ARWSUDQ_RCV_V33_1 (Input), IO8PROG2M25M50M100M_ARWSUDQ_RCV_V33_1_T (Input), IO8PROG2M25M50M100M_I2CIN_RCV_ZII2C_00 (Input), IO8PROG2M25M50M100M_I2CIN_RCV_ZII2C_00_T (Input), IO8PROG2M25M50M100M_I2CIN_RCV_ZII2C_01 (Input), IO8PROG2M25M50M100M_I2CIN_RCV_ZII2C_01_T (Input), IO8PROG2M25M50M100M_I2CIN_RCV_ZII2C_10 (Input), IO8PROG2M25M50M100M_I2CIN_RCV_ZII2C_10_T (Input), IO8PROG2M25M50M100M_I2CIN_RCV_ZII2C_11 (Input), IO8PROG2M25M50M100M_I2CIN_RCV_ZII2C_11_T (Input), IO8PROG2M25M50M100M_I2CIN_RCV_ZIV12_0 (Input), IO8PROG2M25M50M100M_I2CIN_RCV_ZIV12_0_T (Input), IO8PROG2M25M50M100M_I2CIN_RCV_ZIV12_1 (Input), IO8PROG2M25M50M100M_I2CIN_RCV_ZIV12_1_T (Input), IO8PROG2M25M50M100M_I2CIN_RCV_ZIV33_0 (Input), IO8PROG2M25M50M100M_I2CIN_RCV_ZIV33_0_T (Input), IO8PROG2M25M50M100M_I2CIN_RCV_ZIV33_1 (Input), IO8PROG2M25M50M100M_I2CIN_RCV_ZIV33_1_T (Input), IO8USB_ID_OTG_FT_DRV_00 (3-state), IO8USB_ID_OTG_FT_DRV_01 (3-state), IO8USB_ID_OTG_FT_DRV_10 (3-state), IO8USB_ID_OTG_FT_DRV_11 (3-state), IO8USB_ID_OTG_FT_RCV_00 (Input), IO8USB_ID_OTG_FT_RCV_00_T (Input), IO8USB_ID_OTG_FT_RCV_01 (Input), IO8USB_ID_OTG_FT_RCV_01_T (Input)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
